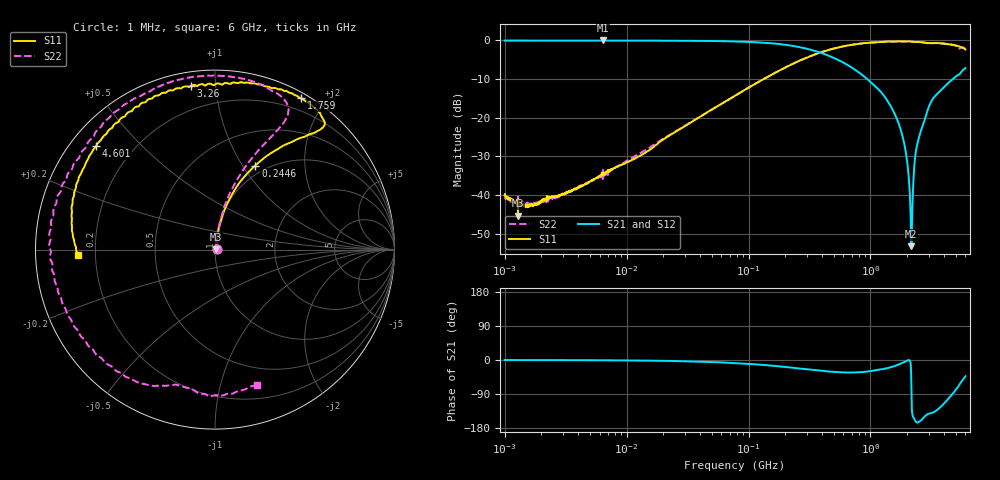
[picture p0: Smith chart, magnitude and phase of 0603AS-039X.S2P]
!s-Parameter Generated by FASTRON Sdn. Bhd.
!FASTRON P/N : 0603AS-039X
!Keysight Technologies: E5071C_MY46733604_B.14.02
!Date: Fri Oct 20 13:30:37 2023
!Version  :Rev01  Fri Oct 20 13:30:37 2023
!Data & Calibration Information:
!Freq  S11:SOLT2(ON)  S21:SOLT2(ON)  S12:SOLT2(ON)  S22:SOLT2(ON)
!PortZ  Port1:50+j0  Port2:50+j0
!When reading reference impedance value at option line is always used.
! Remarks : This data is being provided solely for informational purposes.
# Hz S dB R 50
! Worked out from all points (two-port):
!   1601 points, 1 MHz to 6 GHz, reference 50 ohm
!   highest |S21| = -0.03 dB at 6.378 MHz (marker M1); lowest = -53.2 dB at 2.163 GHz (marker M2)
!   |S21| within 3 dB of the highest: start of sweep to 375.6 MHz
!   lowest |S11| = -45.3 dB at 1.288 MHz (marker M3), VSWR 1.01, Z = 50.5 + j0.181 ohm
!   |S11| at or under -10 dB: start of sweep to 133.3 MHz
!   |S22| runs from -43.0 to -0.3 dB; largest |S21 - S12| = 0.0078
!   S11 on the Smith chart (normalised r, x): 1 MHz: 1.02, +0.01; 244.6 MHz: 0.89, +1.14; 1.759 GHz: 0.06, +1.72; 3.26 GHz: 0.07, +0.86; 4.601 GHz: 0.07, +0.37; 6 GHz: 0.13, -0.02
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1000000  -40.05 17.6  -0.06 -0.1  -0.07 0.0  -40.49 21.3
1287650  -45.31 19.3  -0.07 -0.1  -0.06 -0.1  -39.89 14.7
4277066  -37.73 61.0  -0.07 -0.5  -0.07 -0.5  -37.66 62.0
6378092  -34.66 71.2  -0.03 -0.8  -0.09 -0.8  -35.85 72.3
1.823719e7  -26.55 79.1  -0.08 -2.0  -0.10 -2.0  -26.21 78.1
7.757876e7  -14.32 77.6  -0.27 -8.0  -0.29 -8.0  -14.33 78.9
2.446159e8  -5.69 64.4  -1.58 -21.4  -1.59 -21.4  -5.68 69.0
3.307917e8  -3.93 59.1  -2.52 -26.1  -2.52 -26.0  -3.93 65.4
7.6503e8  -0.97 48.7  -7.81 -32.7  -7.82 -32.6  -0.97 63.0
1.414819e9  -0.32 54.4  -16.21 -20.5  -16.22 -20.5  -0.31 80.6
1.758598e9  -0.27 60.4  -22.84 -10.2  -22.85 -10.2  -0.26 93.0
1.971195e9  -0.29 64.5  -29.98 -2.8  -29.99 -2.8  -0.28 101.2
2.109383e9  -0.30 67.4  -40.79 -2.8  -40.84 -2.9  -0.31 106.6
2.162532e9  -0.36 68.5  -53.21 -63.7  -53.18 -63.1  -0.35 108.7
2.215681e9  -0.36 69.8  -41.04 -146.8  -41.08 -146.7  -0.37 110.9
2.306538e9  -0.40 72.1  -31.12 -157.9  -31.15 -157.8  -0.42 115.0
2.43839e9  -0.43 75.4  -26.38 -164.7  -26.41 -164.7  -0.44 120.6
3.259977e9  -0.70 98.4  -15.04 -138.3  -15.05 -138.3  -0.72 158.6
3.867453e9  -0.82 115.6  -12.59 -119.9  -12.59 -120.2  -0.82 -174.6
4.601007e9  -1.13 138.8  -10.34 -93.4  -10.33 -93.6  -1.13 -140.5
5.272524e9  -1.50 160.0  -8.90 -69.4  -8.90 -69.5  -1.85 -110.0
6e9  -2.35 -177.9  -7.17 -42.8  -7.15 -42.9  -2.07 -72.7
